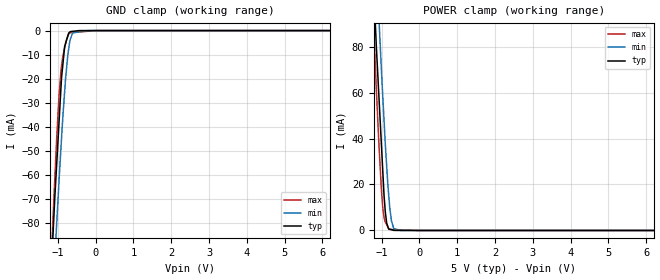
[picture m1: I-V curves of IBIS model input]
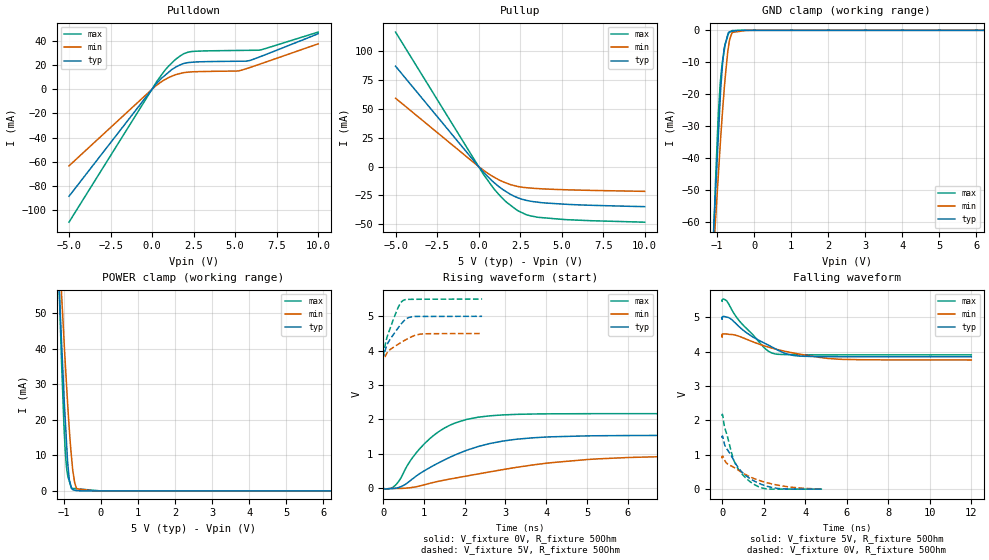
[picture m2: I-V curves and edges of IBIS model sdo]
|Texas Instruments Incorporated
|14-Bit 200KSPS ADC Serial Out, Auto PWRDN, Pseudo Differential Input
| Marketing part#   Digital Voltage Range   Package-type   #pins
| TLC3545ID   4.5V - 5.5V   SOIC   8
| TLC3545IDG4   4.5V - 5.5V   SOIC   8
| TLC3545IDGK   4.5V - 5.5V   MSOP   8
| TLC3545IDGKG4   4.5V - 5.5V   MSOP   8
| TLC3545IDR   4.5V - 5.5V   SOIC   8
| TLC3545IDRG4   4.5V - 5.5V   SOIC   8
[IBIS Ver]   3.2
[File name]   tlc3545.ibs
[File Rev]   1.0
[Date]   12/16/2011
[Source]
| Texas Instruments Incorporated.
| Analog-eLab Design Center, HPA
| 12500 TI Blvd
| Dallas, TX -75243
| e-mail: elab_scm_ibis@list.ti.com
[Notes]   Revision History:
| Rev 1.0: 12/16/2011
| - Initial version of the model
| - Model generated from simulations in TISPICE
| - Model matched to SPICE simulation
| - C_comp although listed in numerical order of value are
|   obtained from varying PVT conditions. For PVT conditions for
|   each specific value refer the buffer description under
|   respective [Model]. IBIS model user is responsible for using
|   appropriate C_comp to simulate for Signal Integrity.
| - Model names with a trailing _5 contains the model for
|   5.0V [4.5V and 5.5V].
[Disclaimer]
| This model is designed as an aid for customers of Texas Instruments.
| TI and its licensors and suppliers make no warranties, either expressed
| or implied, with respect to this  model, including the warranties of
| merchantability or fitness for a particular purpose. The model is
| provided solely on an "as is" basis. The entire risk as to its quality
| and performance is with the customer.
[Copyright]
 (C) Copyright 2011 Texas Instruments Incorporated.All rights reserved.
|   TLC3545D
[Component]   TLC3545D
[Manufacturer]   TI
[Package]   |8 SOIC   -  D package
|   typ   min   max
R_pkg   0.06148   0.03757   0.07125
L_pkg   1.95706nH   1.67767nH   2.20159nH
C_pkg   0.38630pF   0.33316pF   0.43736pF
[Pin]  signal_name   model_name   R_pin   L_pin   C_pin
1   _CS   input   0.06879   2.15059nH  0.40544pF
2   REF   term   0.06164   1.67767nH  0.33316pF
3   GND   gnd   0.02421   1.44903nH  0.39057pF
4   AIN(+)   term   0.06655   2.11510nH  0.40019pF
5   AIN(-)   term   0.03757   1.89090nH  0.43736pF
6   VDD   power   0.03556   1.48930nH  0.37852pF
7   SCLK   input   0.06308   1.70652nH  0.33444pF
8   SDO   sdo   0.07125   2.20159nH  0.40720pF
|   TLC3545DGK
[Component]   TLC3545DGK
[Manufacturer]   TI
[Package]   |8 MSOP   -  DGK package
|   typ   min   max
R_pkg   0.04462   0.02664   0.04990
L_pkg   1.43112nH   1.25021nH   1.50284nH
C_pkg   0.37756pF   0.36322pF   0.39650pF
[Pin]  signal_name   model_name   R_pin   L_pin   C_pin
1   _CS   input   0.04860   1.47792nH  0.36540pF
2   REF   term   0.04815   1.46022nH  0.38825pF
3   GND   gnd   0.01822   1.20018nH  0.42710pF
4   AIN(+)   term   0.04786   1.46638nH  0.36322pF
5   AIN(-)   term   0.02664   1.25021nH  0.39650pF
6   VDD   power   0.02611   1.23843nH  0.41737pF
7   SCLK   input   0.04659   1.42918nH  0.38607pF
8   SDO   sdo   0.04990   1.50284nH  0.36595pF
[Model] term
Model_type Terminator
C_comp   1.0e-20F  1.0e-20F  1.0e-20F
|   typ   min   max
[Voltage Range]   5.0V   4.5V   5.5V
[POWER Clamp Reference]   5.0V   4.5V   5.5V
[GND Clamp Reference]   0V   0V   0V
|Ambient Temperature   25   85   -40
|Junction Temperature
[Temperature Range]   27   125   -40
| Models and submodels in the file (3): input (Input), sdo (3-state), term (Terminator)
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|   input Model
[Model]   input
Model_type   Input
Vinl = 0.8
Vinh = 2.1
|   typ   min   max
 C_comp   8.474e-13   8.443e-13   8.631e-13
| Where nom  PVT is Nominal Process, 5V, 27C
|   Fast PVT is Strong Process,  5.5V, -40C
|   Slow PVT is Weak Process,   4.5V, 125C
[Voltage Range]   5   4.5   5.5
|Ambient Temperature   25   85   -40
|Junction Temperature
[Temperature Range]   27   125   -40
[Power Clamp Reference]   5   4.5   5.5
[GND Clamp Reference]   0   0   0
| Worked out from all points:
|   GND clamp passes 1 mA (typ) near -0.71 V on its own axis
|   POWER clamp passes 1 mA (typ) near -0.82 V on its own axis
[GND Clamp]
|   Voltage   I(typ)   I(min)   I(max)
-5V       -1.642A    -1.556A    -1.737A
-1.14V    -88.6mA    -113.3mA   -82.6mA
-1.122V   -82.8mA    -107.6mA   -75.77mA
-1.034V   -56.4mA    -81.18mA   -45.82mA
-973.5mV  -39.47mA   -63.79mA   -28.29mA
-918.5mV  -24.09mA   -48.91mA   -16.95mA
-820mV    -6.626mA   -25.32mA   -7.129mA
-738mV    -2.306mA   -10.42mA   -2.484mA
-670mV    -434.4uA   -3.583mA   -913.3uA
-607.5mV  -319.1uA   -935.8uA   -828.1uA
-202.5mV  -317.6nA   -25.16nA   -276uA
10V       0A         0A         0A
[POWER Clamp]
|   Voltage   I(typ)   I(min)   I(max)
-5V       1.659A     1.659A     1.672A
-1.373V   166.8mA    201.2mA    150.9mA
-1.14V    80.35mA    116.4mA    61.93mA
-1.062V   55.39mA    89.15mA    34.63mA
-968mV    25.65mA    58.09mA    9.832mA
-905mV    8.771mA    38.6mA     3.843mA
-865mV    3.188mA    27.92mA    2.517mA
-803mV    642uA      13.67mA    460.9uA
-738mV    336.8uA    4.073mA    423.6uA
-679.5mV  62.11uA    957.2uA    390uA
-486mV    8.246uA    4.552uA    278.9uA
10V       0A         0A         0A
|   sdo Model
[Model]   sdo
Model_type   3-state
Polarity   Non-Inverting
Vmeas = 2.5
Vref = 2.5
Cref = 2pF
Rref = 50
|   typ   min   max
|   (nom PVT)   (fast PVT)   (slow PVT)
 C_comp   2.635e-12   2.372e-12   3.010e-12
| Where nom  PVT is Nominal Process, 5V, 27C
|   Fast PVT is Strong Process,  5.5V, -40C
|   Slow PVT is Weak Process,   4.5V, 125C
[Voltage Range]   5   4.5   5.5
|Ambient Temperature   25   85   -40
|Junction Temperature
[Temperature Range]   27   125   -40
[Pullup Reference]   5   4.5   5.5
[Pulldown Reference]   0   0   0
[Power Clamp Reference]   5   4.5   5.5
[GND Clamp Reference]   0   0   0
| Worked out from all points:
|   slope of the pulldown table from 0 to 0.75 V, typ, clamps not added: 67.3 ohm
|   slope of the pullup table from 0 to 0.75 V, typ, clamps not added: 65.5 ohm
|   GND clamp passes 1 mA (typ) near -0.70 V on its own axis
|   POWER clamp passes 1 mA (typ) near -0.80 V on its own axis
|   falling waveform, V_fixture 5V, R_fixture 50Ohm: 20-80 % time 1.83ns typ, 2.73ns min, 1.36ns max; typ from 5 V to 3.85 V
|   rising waveform, V_fixture 0V, R_fixture 50Ohm: 20-80 % time 1.62ns typ, 2.95ns min, 989ps max; typ from 0 V to 1.54 V
|   rising waveform, V_fixture 5V, R_fixture 50Ohm: 20-80 % time 369ps typ, 523ps min, 280ps max; typ from 3.85 V to 5 V
|   falling waveform, V_fixture 0V, R_fixture 50Ohm: 20-80 % time 1.18ns typ, 1.92ns min, 817ps max; typ from 1.54 V to 0 V
[Pulldown]
|   Voltage   I(typ)   I(min)   I(max)
-5V       -88.35mA   -63.24mA   -109.7mA
297mV     5.075mA    3.491mA    6.673mA
797.5mV   11.69mA    8.128mA    16.01mA
1.205V    16.38mA    10.88mA    21.88mA
1.485V    18.7mA     12.3mA     25.38mA
1.925V    21.31mA    13.75mA    29.41mA
2.376V    22.24mA    14.35mA    31.13mA
5.193V    23.12mA    15.11mA    32.03mA
5.9V      23.75mA    17.97mA    32.13mA
6.6V      27.34mA    21.26mA    32.7mA
10V       45.81mA    37.47mA    47.18mA
[GND Clamp]
|   Voltage   I(typ)   I(min)   I(max)
-5V       -1.331A    -1.082A    -1.684A
-1.089V   -61.38mA   -67.85mA   -62.28mA
-1.034V   -48.66mA   -57.7mA    -44.65mA
-968mV    -33.39mA   -45.51mA   -26.62mA
-907.5mV  -19.4mA    -34.35mA   -15.41mA
-855mV    -10.71mA   -25.55mA   -9.671mA
-810mV    -5.627mA   -18.69mA   -6.502mA
-775.5mV  -4.12mA    -14.04mA   -4.073mA
-711mV    -1.304mA   -6.62mA    -1.706mA
-657mV    -414.4uA   -2.687mA   -588.6uA
-594mV    -297uA     -671.1uA   -61.03uA
10V       0A         0A         0A
[Pullup]
|   Voltage   I(typ)   I(min)   I(max)
-5V       87.04mA    59.28mA    116.6mA
286mV     -4.7mA     -3.047mA   -6.573mA
880mV     -13.25mA   -8.731mA   -18.48mA
1.238V    -17.55mA   -11.61mA   -24.52mA
1.672V    -21.84mA   -14.26mA   -30.76mA
2.283V    -26.55mA   -16.96mA   -37.51mA
2.871V    -29.27mA   -18.3mA    -41.7mA
3.591V    -30.92mA   -19.08mA   -43.99mA
5.192V    -32.6mA    -20.06mA   -45.95mA
10V       -34.72mA   -21.47mA   -48.2mA
[POWER Clamp]
|   Voltage   I(typ)   I(min)   I(max)
-5V       1.167A     980.3mA    1.513A
-1.133V   58.35mA    69.23mA    58.01mA
-1.062V   41.15mA    54.8mA     35.46mA
-1.001V   27.3mA     42.93mA    18.81mA
-962.5mV  19.62mA    35.67mA    10.81mA
-905mV    8.826mA    25.39mA    4.74mA
-855mV    3.125mA    17.31mA    2.702mA
-765mV    381uA      6.073mA    709uA
-711mV    207uA      2.355mA    658.9uA
-648mV    67.94uA    584.3uA    600.5uA
-202.5mV  96.37nA    0A         187.7uA
10V       0A         0A         0A
[Ramp]
R_load = 50
|   typ   min   max
dV/dt_r   0.922171/1.61922e-09   0.571123/2.9559e-09   1.30126/9.88725e-10
dV/dt_f   0.68885/1.8285e-09   0.444423/2.72741e-09   0.954632/1.35814e-09
[Falling Waveform]
V_fixture = 5V
V_fixture_min = 4.5V
V_fixture_max = 5.5V
R_fixture = 50Ohm
|   Time   V(typ)   V(min)   V(max)
0s        5V         4.5V       5.5V
2ps       4.943V     4.423V     5.465V
26ps      5.018V     4.511V     5.524V
220ps     5.008V     4.516V     5.479V
788ps     4.747V     4.456V     4.927V
1.98ns    4.266V     4.18V      4.143V
2.548ns   4.09V      4.081V     3.936V
3.438ns   3.891V     3.962V     3.913V
5.73ns    3.853V     3.778V     3.909V
12ns      3.852V     3.759V     3.909V
[Rising Waveform]
V_fixture = 0V
V_fixture_min = 0V
V_fixture_max = 0V
R_fixture = 50Ohm
|   Time   V(typ)   V(min)   V(max)
0s        3.118nV    3.515nV    3.001nV
314ps     1.884mV    -6.242mV   102.9mV
764ps     310.9mV    33.69mV    956.9mV
1.2ns     636.7mV    159.7mV    1.498V
1.646ns   905.3mV    269.2mV    1.836V
2.048ns   1.104V     355.5mV    2.001V
2.938ns   1.371V     542.6mV    2.131V
3.982ns   1.488V     724mV      2.162V
6.032ns   1.532V     894.6mV    2.168V
9.066ns   1.537V     946mV      2.169V
[Rising Waveform]
V_fixture = 5V
V_fixture_min = 4.5V
V_fixture_max = 5.5V
R_fixture = 50Ohm
|   Time   V(typ)   V(min)   V(max)
0s        3.852V     3.759V     3.909V
2ps       3.903V     3.835V     3.936V
20ps      3.864V     3.753V     3.948V
102ps     4.184V     3.943V     4.409V
290ps     4.531V     4.126V     5.027V
412ps     4.729V     4.216V     5.351V
504ps     4.856V     4.282V     5.466V
648ps     4.968V     4.375V     5.491V
984ps     4.994V     4.487V     5.493V
2.428ns   4.997V     4.496V     5.499V
[Falling Waveform]
V_fixture = 0V
V_fixture_min = 0V
V_fixture_max = 0V
R_fixture = 50Ohm
|   Time   V(typ)   V(min)   V(max)
0s        1.537V     952.8mV    2.169V
28ps      1.531V     960.6mV    2.147V
102ps     1.338V     868.3mV    1.847V
162ps     1.233V     796.8mV    1.712V
590ps     807.8mV    623.7mV    799.8mV
828ps     583.3mV    534.6mV    538.1mV
1.348ns   304.8mV    356.1mV    215.9mV
1.976ns   119.7mV    216.9mV    24.77mV
2.67ns    21.28mV    116.2mV    104.7uV
4.812ns   265uV      2.041mV    200.7uV
